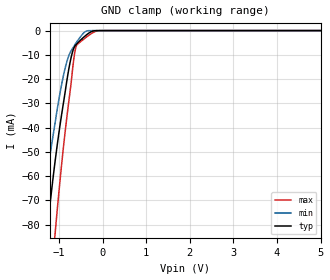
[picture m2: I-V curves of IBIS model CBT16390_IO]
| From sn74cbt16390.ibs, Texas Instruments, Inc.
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[Model]   CBT16390_IO
Model_type  Terminator
| variable   typ   min   max
C_comp   4.64pF   3.68pF   6.27pF
| C_tri-state   4.64pF   3.68pF   6.27pF
[Temperature Range]   40   100   -40
| Ambient temperature   25   85   -40
[Voltage range]   5   4.5   5.5
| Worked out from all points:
|   GND clamp passes 1 mA (typ) near -0.31 V on its own axis
[GND Clamp]
| CBT16390_IO
|   Voltage   I(typ)   I(min)   I(max)
-5V       -918.1mA   -821.9mA   -1.124A
-1.435V   -112.7mA   -83.49mA   -161.8mA
-1.28V    -84.27mA   -60.84mA   -125.3mA
-1.09V    -54.02mA   -38.12mA   -83.88mA
-965mV    -37.63mA   -24.62mA   -59.75mA
-855mV    -24.85mA   -15.19mA   -41.15mA
-735mV    -12.16mA   -8.733mA   -23.54mA
-645mV    -6.677mA   -6.104mA   -9.749mA
-595mV    -5.551mA   -4.736mA   -5.998mA
-395mV    -2.125mA   -418.6uA   -3.004mA
-90mV     -2.483uA   -3.944nA   -61.87uA
5V        333.5nA    371.2pA    4.468uA
